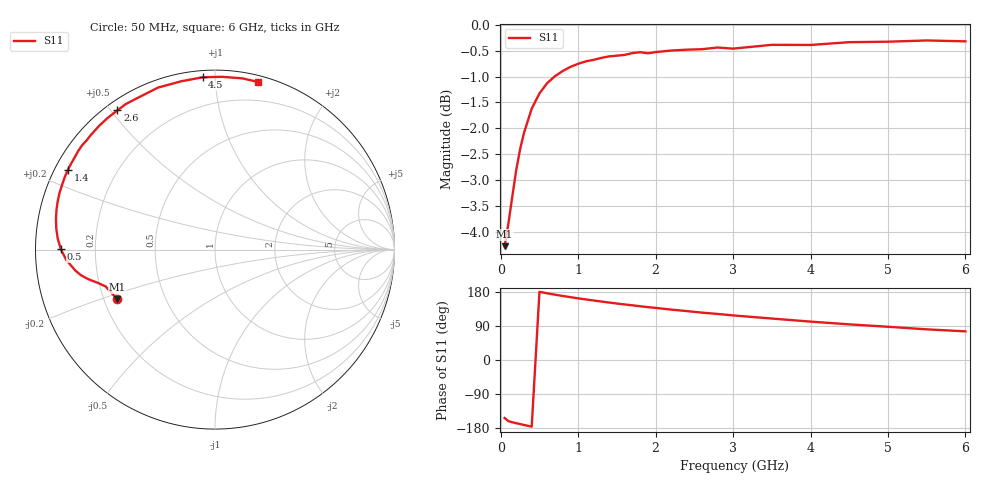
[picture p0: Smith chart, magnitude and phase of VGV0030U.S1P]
! Infineon Technologies  Discrete & RF Semiconductors
! BB 831
! Si Tuning Diode in SOD323
! VR =
! S-Parameters:  July  1999
# GHz  S  MA  R  50
!  f  S11
! GHz  MAG  ANG
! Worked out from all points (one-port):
!   34 points, 50 MHz to 6 GHz, reference 50 ohm
!   lowest |S11| = -4.3 dB at 50 MHz (marker M1), VSWR 4.14, Z = 12.7 - j11.2 ohm
!   |S11| at or under -10 dB: nowhere
!   S11 on the Smith chart (normalised r, x): 50 MHz: 0.25, -0.22; 500 MHz: 0.08, +0.00; 1.4 GHz: 0.04, +0.25; 2.6 GHz: 0.03, +0.52; 4.5 GHz: 0.04, +0.93; 6 GHz: 0.05, +1.29
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0.05  0.6107 -153.1
0.1  0.6431 -161.4
0.2  0.7238 -166.8
0.25  0.7581 -169.0
0.3  0.7861 -171.4
0.4  0.8298 -175.9
0.5  0.8586 179.9
0.6  0.8785 176.0
0.7  0.8922 172.4
0.8  0.9025 169.0
0.9  0.9109 165.8
1.1  0.9222 159.8
1.4  0.9325 151.6
1.6  0.9355 146.6
1.7  0.9393 144.3
1.9  0.9389 139.5
2  0.9414 137.5
2.2  0.9446 133.0
2.4  0.9465 129.1
2.6  0.9475 125.0
2.8  0.9511 121.5
3  0.9487 117.7
3.5  0.9568 109.4
4  0.9565 101.3
4.5  0.9625 94.1
5  0.9635 87.7
5.5  0.9662 80.9
6  0.9643 75.6
